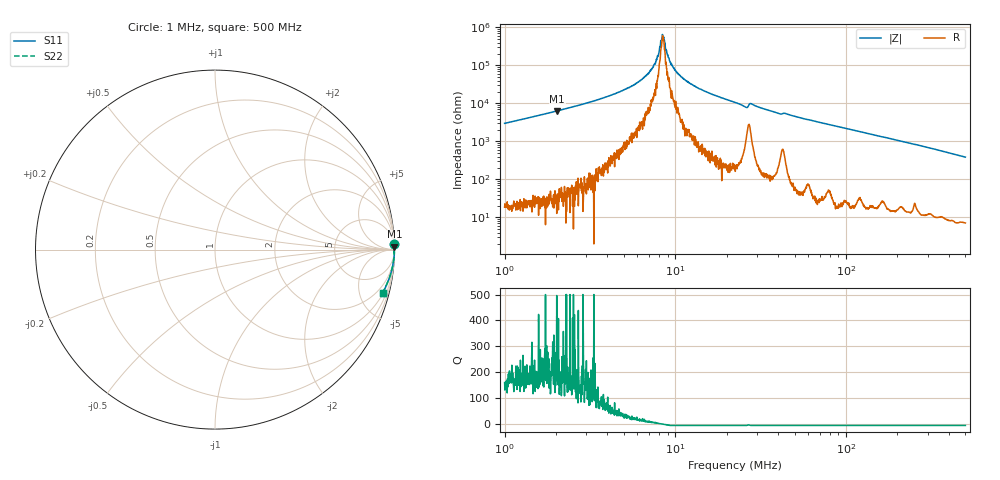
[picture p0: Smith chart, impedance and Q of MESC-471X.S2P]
!s-Parameter Generated by FASTRON Sdn. Bhd.
!FASTRON P/N : MESC-471X
!Keysight Technologies,E4991B,MY54100416,A.01.15
!Date: Fri Mar 27 11:43:03 2026
!Version  : Rev00 Fri Mar 27 11:43:03 2026
!Data & Calibration Information:
!PortZ  Port1:50+j0  Port2:50+j0
!When reading, reference impedance value at option line is always used.
! Remarks : This data is being provided solely for informational purposes.
!Freq	S11	S21	S12	S22
# Hz S dB R 50
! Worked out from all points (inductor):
!   1601 points, 1 MHz to 500 MHz, reference 50 ohm
!   read as one part in series: L = 471 uH near 1.032 MHz
!   highest Q = 260 at 2.036 MHz (marker M1), where L = 500 uH
!   self-resonance near 8.435 MHz
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1000000  -0.01 1.9  -29.54 -87.7  -29.54 -87.7  -0.01 1.9
2035611  -0.00 0.9  -36.11 -88.8  -36.11 -88.8  -0.00 0.9
2820919  -0.00 0.6  -39.44 -89.1  -39.44 -89.1  -0.00 0.6
4307824  -0.00 0.3  -44.75 -88.4  -44.75 -88.4  -0.00 0.3
5877687  -0.00 0.2  -50.56 -87.0  -50.56 -87.0  -0.00 0.2
7193214  -0.00 0.1  -57.79 -83.6  -57.79 -83.6  -0.00 0.1
7595196  -0.00 0.0  -61.14 -78.3  -61.14 -78.3  -0.00 0.0
7957584  -0.00 0.0  -65.65 -74.0  -65.65 -74.0  -0.00 0.0
8304943  -0.00 0.0  -73.17 -45.5  -73.17 -45.5  -0.00 0.0
8467807  -0.00 -0.0  -75.47 5.9  -75.47 5.9  -0.00 -0.0
8667465  -0.00 -0.0  -71.16 44.8  -71.16 44.8  -0.00 -0.0
9045811  -0.00 -0.0  -65.46 75.8  -65.46 75.8  -0.00 -0.0
9514295  -0.00 -0.1  -60.76 78.4  -60.76 78.4  -0.00 -0.1
1.098475e7  -0.00 -0.1  -53.63 86.5  -53.63 86.5  -0.00 -0.1
1.392158e7  -0.00 -0.2  -47.67 88.3  -47.67 88.3  -0.00 -0.2
2.236068e7  -0.00 -0.5  -40.57 88.2  -40.57 88.2  -0.00 -0.5
2.581658e7  -0.01 -0.7  -38.08 82.5  -38.08 82.5  -0.01 -0.7
2.801062e7  -0.01 -0.6  -39.78 83.0  -39.78 83.0  -0.01 -0.6
4.035405e7  -0.01 -1.0  -34.75 86.5  -34.75 86.5  -0.01 -1.0
6.307767e7  -0.01 -1.6  -31.06 87.8  -31.06 87.8  -0.01 -1.6
1.77937e8  -0.04 -4.7  -21.73 84.5  -21.73 84.5  -0.04 -4.7
5e8  -0.32 -14.4  -12.08 74.5  -12.08 74.5  -0.32 -14.4
